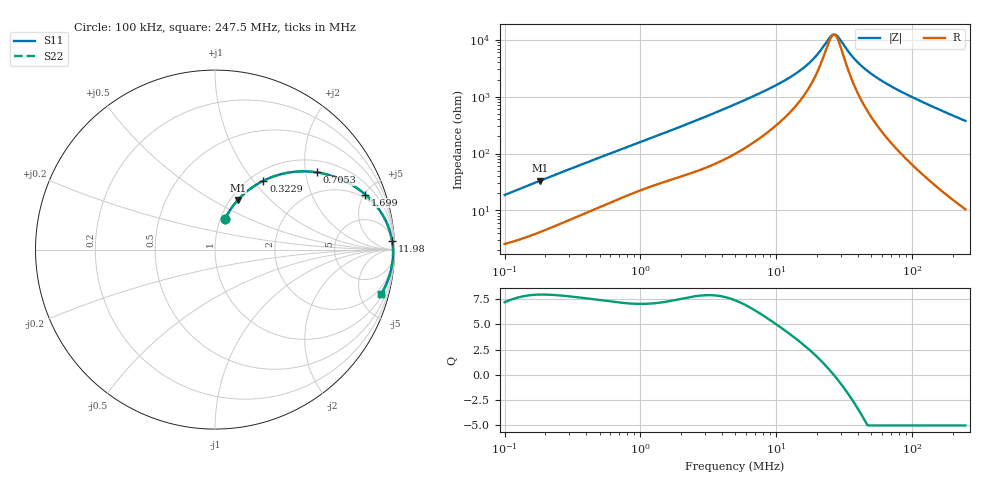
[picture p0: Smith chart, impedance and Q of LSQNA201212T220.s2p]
! LSQNA201212T220  S-PARAMETER MODEL  ( General Type )
! Model Generated by TAIYO YUDEN Corporation (http://www.ty-top.com)
! Version 2.0
! TAIYO YUDEN Control No. 100810NF25SB-FKC
! Copyright(c) 2007 TAIYO YUDEN CO.,LTD. All Rights Reserved.
! Product Description (link to TY-COMPAS)
! https://ds.yuden.co.jp/TYCOMPAS/or/detail?pn=LSQNA201212T220K&u=M
! Products Name : Inductors
! Characteristics :
!  Inductance : 22 uH , SRF(min) : 16 MHz , DC Resistance(max) : 2.21 Ohm
!  Rated Current : Saturation :135 mA , Temp Rise : 280 mA (40 degC)
!  Case Size : 2.0 x 1.25 / 0.079 x 0.049 [mm/inch] , Thickness : 1.25 / 0.049 [mm/inch]
!  (Conditions: Temperature = 25 degC , DC Bias Current/Voltage = 0A / 0V)
! External Node Assignments :
!  1  o---GGG---o  2
! GND o---------o GND
! Frequency Range : 0.1MHz  -  247.502633MHz  [ 402 STEP ]
# MHz S RI R 50
! Freq[MHz].  S11 Real  S11 Imag  S21 Real  S21 Imag  S12 Real  S12 Imag  S22 Real  S22 Imag
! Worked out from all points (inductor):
!   401 points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, 100 kHz to 247.5 MHz, reference 50 ohm
!   read as one part in series: L = 29.2 uH near 104 kHz
!   highest Q = 7.93 at 183.2 kHz (marker M1), where L = 28.8 uH
!   self-resonance near 26.18 MHz
!   S11 on the Smith chart (normalised r, x): 100 kHz: 1.05, +0.37; 322.9 kHz: 1.15, +1.13; 705.3 kHz: 1.32, +2.30; 1.699 MHz: 1.70, +5.11; 11.98 MHz: 10, +39; 247.5 MHz: 1.21, -7.48
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0.1  0.0558 0.1702  0.9442 -0.1702  0.9442 -0.1702  0.0558 0.1702
0.183232  0.1283 0.2773  0.8717 -0.2773  0.8717 -0.2773  0.1283 0.2773
0.322877  0.2692 0.3834  0.7308 -0.3834  0.7308 -0.3834  0.2692 0.3834
0.37019  0.3152 0.4036  0.6848 -0.4036  0.6848 -0.4036  0.3152 0.4036
0.705334  0.5658 0.4305  0.4342 -0.4305  0.4342 -0.4305  0.5658 0.4305
1.370406  0.7869 0.3453  0.2131 -0.3453  0.2131 -0.3453  0.7869 0.3453
1.698919  0.8383 0.3062  0.1617 -0.3062  0.1617 -0.3062  0.8383 0.3062
2.768671  0.9189 0.2165  0.0811 -0.2165  0.0811 -0.2165  0.9189 0.2165
4.974964  0.9649 0.1283  0.0351 -0.1283  0.0351 -0.1283  0.9649 0.1283
8.267469  0.9809 0.0752  0.0191 -0.0752  0.0191 -0.0752  0.9809 0.0752
11.98306  0.9866 0.0469  0.0134 -0.0469  0.0134 -0.0469  0.9866 0.0469
15.14869  0.9889 0.0319  0.0111 -0.0319  0.0111 -0.0319  0.9889 0.0319
18.41681  0.9903 0.0205  0.00968 -0.0205  0.00968 -0.0205  0.9903 0.0205
25.17432  0.9918 0.00298  0.00819 -0.00298  0.00819 -0.00298  0.9918 0.00298
27.22034  0.992 -0.00137  0.00796 0.00137  0.00796 0.00137  0.992 -0.00137
28.86326  0.9922 -0.00466  0.00783 0.00466  0.00783 0.00466  0.9922 -0.00466
35.09012  0.9924 -0.0159  0.00762 0.0159  0.00762 0.0159  0.9924 -0.0159
41.83506  0.9922 -0.0266  0.00778 0.0266  0.00778 0.0266  0.9922 -0.0266
51.86374  0.9915 -0.0409  0.0085 0.0409  0.0085 0.0409  0.9915 -0.0409
68.1772  0.9895 -0.0618  0.0105 0.0618  0.0105 0.0618  0.9895 -0.0618
120.1361  0.9784 -0.1212  0.0216 0.1212  0.0216 0.1212  0.9784 -0.1212
247.5026  0.9273 -0.246  0.0727 0.246  0.0727 0.246  0.9273 -0.246
